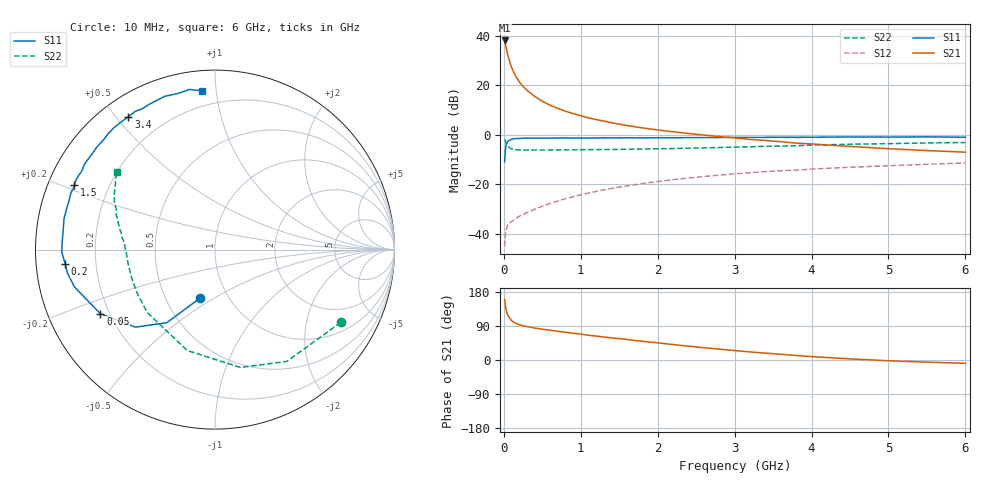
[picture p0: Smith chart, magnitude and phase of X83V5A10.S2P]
! SIEMENS Small Signal Semiconductors
! BFP136W
! Si NPN RF Bipolar Junction Transistor in SOT343
! VCE = 3.5 V  IC = 100 mA
! Common Emitter S-Parameters:  September  1994
# GHz  S  MA  R  50
!  f  S11  S21  S12  S22
! GHz  MAG  ANG  MAG  ANG  MAG  ANG  MAG  ANG
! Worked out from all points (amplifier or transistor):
!   40 points, 10 MHz to 6 GHz, reference 50 ohm
!   highest |S21| = 38.1 dB at 10 MHz (marker M1)
!   |S21| within 3 dB of that: start of sweep to 31.32 MHz
!   unconditionally stable (mu >= 1): 533.7 MHz to 2.887 GHz
!   at 200 MHz: K = 0.68, MSG = 27.2 dB, |S12| = -33.0 dB
!   at 1.5 GHz: K = 1.10, MAG = 10.8 dB, |S12| = -21.2 dB
!   at 6 GHz: K = 0.97, MSG = 2.2 dB, |S12| = -11.4 dB
!   S11 on the Smith chart (normalised r, x): 10 MHz: 0.74, -0.43; 50 MHz: 0.17, -0.25; 200 MHz: 0.09, -0.05; 1.5 GHz: 0.08, +0.22; 3.4 GHz: 0.08, +0.54; 6 GHz: 0.11, +0.92
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0.01  0.2821 -107.0  79.99 160.2  0.0056 69.3  0.8099 -30.0
0.02  0.4879 -123.4  68.61 143.9  0.0092 58.3  0.7404 -57.3
0.03  0.6197 -135.8  57.91 132.2  0.0119 49.4  0.6718 -77.8
0.05  0.7319 -150.8  41.32 118.1  0.015 39.6  0.583 -105.4
0.1  0.8108 -165.2  22.85 103.6  0.0177 37.4  0.5151 -137.3
0.15  0.8332 -171.2  15.57 97.2  0.0201 39.8  0.4967 -150.6
0.2  0.8389 -174.6  11.69 93.2  0.0225 41.4  0.4915 -157.8
0.25  0.8477 -177.5  9.436 90.3  0.0245 44.0  0.4905 -162.4
0.3  0.8539 -179.2  7.893 88.2  0.0267 47.0  0.4887 -165.5
0.4  0.8526 177.2  5.944 84.4  0.0312 51.0  0.4898 -169.7
0.5  0.8519 174.4  4.739 81.2  0.0359 54.3  0.4905 -172.5
0.6  0.8527 172.6  3.953 78.7  0.0407 56.1  0.4914 -174.4
0.7  0.8562 169.8  3.411 75.6  0.0458 58.1  0.4927 -175.8
0.9  0.8572 166.6  2.668 70.6  0.0557 59.7  0.4948 -178.4
1.1  0.8573 161.9  2.184 65.3  0.0661 60.3  0.4985 179.9
1.5  0.8618 155.3  1.627 56.3  0.0874 59.8  0.505 176.8
2.2  0.8676 143.1  1.142 40.8  0.1232 54.9  0.5248 171.4
3.2  0.8828 126.2  0.804 21.3  0.1702 45.7  0.5689 162.6
3.4  0.8832 123.1  0.763 18.1  0.1798 43.6  0.5822 160.9
4.5  0.8988 108.0  0.578 2.9  0.2198 33.5  0.6406 151.2
5.5  0.9033 99.0  0.478 -5.7  0.2525 25.7  0.6804 144.5
6  0.8878 94.6  0.443 -8.7  0.2684 21.3  0.6951 141.5
